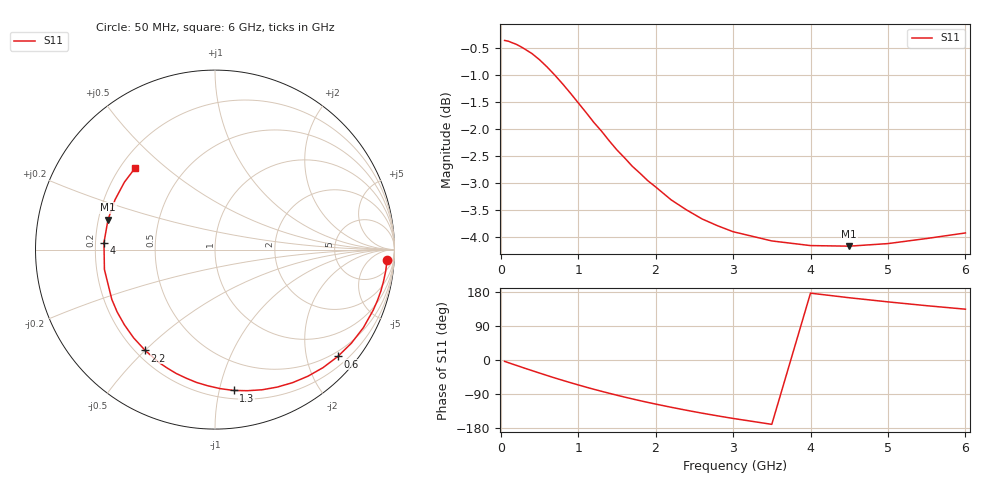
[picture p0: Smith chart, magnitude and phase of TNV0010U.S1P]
! SIEMENS Discrete & RF Semiconductors
! BAS70-07W
! Si Schottky Diode in SOT343
! IF = 0.01 mA
! S-Parameters:  February  1997
# GHz  S  MA  R  50
!  f  S11
! GHz  MAG  ANG
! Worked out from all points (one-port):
!   34 points, 50 MHz to 6 GHz, reference 50 ohm
!   lowest |S11| = -4.2 dB at 4.5 GHz (marker M1), VSWR 4.25, Z = 12 + j6.51 ohm
!   |S11| at or under -10 dB: nowhere
!   S11 on the Smith chart (normalised r, x): 50 MHz: 15, -22; 600 MHz: 0.39, -2.62; 1.3 GHz: 0.26, -1.11; 2.2 GHz: 0.24, -0.50; 4 GHz: 0.23, +0.03; 6 GHz: 0.26, +0.40
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0.05  0.9603 -3.6
0.2  0.9525 -14.1
0.3  0.9438 -21.0
0.4  0.9341 -27.7
0.5  0.9217 -34.4
0.6  0.9072 -41.0
0.7  0.8916 -47.5
0.8  0.8751 -53.7
0.9  0.8581 -59.8
1  0.8407 -65.7
1.1  0.8237 -71.5
1.3  0.7915 -82.5
1.4  0.7752 -87.8
1.6  0.7474 -97.9
1.8  0.7231 -107.4
1.9  0.7118 -111.9
2  0.7025 -116.3
2.2  0.6834 -124.7
2.4  0.6688 -132.7
2.6  0.6561 -140.3
2.8  0.6466 -147.4
3  0.6385 -154.2
3.5  0.626 -169.8
4  0.6198 176.4
4.5  0.619 164.3
5  0.6225 153.4
5.5  0.6293 143.3
6  0.6368 134.1
